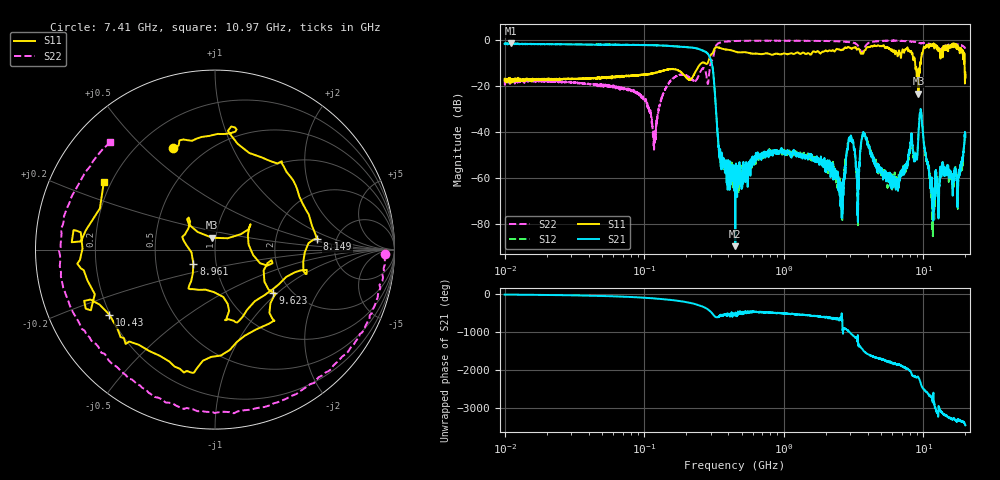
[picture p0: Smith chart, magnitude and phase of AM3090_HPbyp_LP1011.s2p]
# Hz S DB R 50
!freq MagS11 AngS11 MagS21 AngS21 MagS12 AngS12 MagS22 AngS22
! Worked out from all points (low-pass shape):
!   3201 points, 10 MHz to 20 GHz, reference 50 ohm
!   highest |S21| = -1.46 dB at 11.1 MHz (marker M1); lowest = -89.8 dB at 449.3 MHz (marker M2)
!   |S21| within 3 dB of the highest: start of sweep to 259.4 MHz
!   lowest |S11| = -23.3 dB at 9.22 GHz (marker M3), VSWR 1.15, Z = 48 + j6.37 ohm
!   |S11| at or under -10 dB: start of sweep to 257.8 MHz; 8.728 GHz to 9.474 GHz (747 MHz wide, 8.21 % of centre); 19.73 GHz to end of sweep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
!   |S22| runs from -47.8 to -0.2 dB; largest |S21 - S12| = 0.033
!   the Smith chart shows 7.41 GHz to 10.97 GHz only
!   S11 on the Smith chart (normalised r, x): 7.41 GHz: 0.34, +0.61; 8.149 GHz: 3.56, +0.64; 8.961 GHz: 0.78, -0.13; 9.623 GHz: 1.62, -0.94; 10.43 GHz: 0.20, -0.27; 10.97 GHz: 0.17, +0.27
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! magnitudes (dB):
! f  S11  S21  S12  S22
! 10 MHz  -17.4  -1.7  -1.7  -17.7
! 11.1 MHz  -18.0  -1.5  -1.7  -17.8
! 35.55 MHz  -16.7  -2.0  -1.9  -18.9
! 126.1 MHz  -13.9  -2.3  -2.3  -31.5
! 289.6 MHz  -9.0  -6.5  -6.4  -17.1
! 351.8 MHz  -3.5  -51.7  -53.0  -1.1
! 447.2 MHz  -5.0  -58.3  -58.1  -0.4
! 449.3 MHz  -5.0  -89.8  -57.2  -0.4
! 1.59 GHz  -5.7  -50.9  -50.0  -0.3
! 2.575 GHz  -4.5  -64.4  -72.7  -0.6
! 2.962 GHz  -3.4  -43.8  -43.1  -0.9
! 3.384 GHz  -3.8  -70.7  -68.4  -2.3
! 3.775 GHz  -4.6  -41.3  -41.3  -3.6
! 5.639 GHz  -3.7  -61.7  -61.9  -0.3
! 7.41 GHz  -4.3  -55.4  -56.3  -0.5
! 8.149 GHz  -4.8  -42.5  -44.2  -0.7
! 8.961 GHz  -16.8  -50.9  -51.7  -0.9
! 9.22 GHz  -23.3  -41.0  -41.3  -1.0
! 9.623 GHz  -7.9  -31.1  -31.3  -1.4
! 10.43 GHz  -3.2  -50.0  -50.6  -1.3
! 10.97 GHz  -2.8  -56.8  -54.9  -1.5
! 20 GHz  -14.2  -42.3  -40.4  -3.7
